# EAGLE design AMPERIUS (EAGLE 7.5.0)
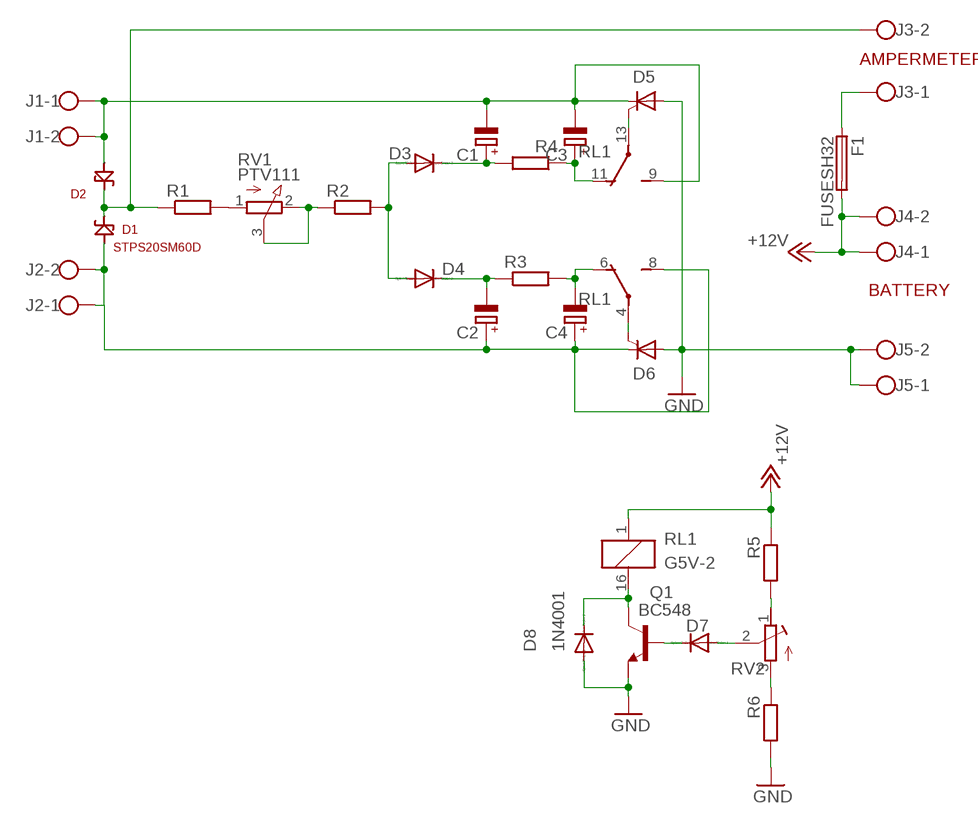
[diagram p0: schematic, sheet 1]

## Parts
C1  CPOL-EUE2.5-7  [E2,5-7]
C2  CPOL-EUE2.5-7  [E2,5-7]
C3  CPOL-EUE2.5-7  [E2,5-7]
C4  CPOL-EUE2.5-7  [E2,5-7]
D1  STPS20SM60D  [TO-220-2]
D2  STPS20SM60D  [TO-220-2]
D3  1N4148DO35-10  [DO35-10]
D4  1N4148DO35-10  [DO35-10]
D5  BTW58  [TO220CS]
D6  BTW58  [TO220CS]
D7  1N4148DO35-10  [DO35-10]
D8  1N4001  1N4004  [DO41-10]
F1  FUSESH32  [SH32]
J1  W237-102  [W237-102]
J2  W237-102  [W237-102]
J3  W237-102  [W237-102]
J4  W237-102  [W237-102]
J5  W237-102  [W237-102]
Q1  BC548  [TO92-EBC]
R1  R-EU_0207/10  [0207/10]
R2  R-EU_0207/10  [0207/10]
R3  R-EU_0207/10  [0207/10]
R4  R-EU_0207/10  [0207/10]
R5  R-EU_0207/10  [0207/10]
R6  R-EU_0207/10  [0207/10]
RL1  G5V-2  [G5V-2]
RV1  PTV111  [PTV111]
RV2  R-TRIMM-3386-F  [R-TRIMM-3386F]

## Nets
+12V: F1.2A J4.1 J4.2 R5.1 RL1.1
GND: D5.A D6.A D8.A J5.1 J5.2 Q1.E R6.2
N$1: D1.1(K) D2.1(K) J3.2 R1.1
N$2: C1.- C3.- D2.3(A) D5.C J1.1 J1.2 RL1.9(2:S)
N$3: C2.+ C4.+ D1.3(A) D6.C J2.1 J2.2 RL1.8(1:S)
N$4: R1.2 RV1.1(A)
N$5: R2.1 RV1.2(E) RV1.3(S)
N$6: D3.A D4.A R2.2
N$7: C1.+ D3.C R4.2
N$8: C2.- D4.C R3.1
N$9: F1.1A J3.1
N$10: D5.G RL1.13(2:P)
N$11: C4.- R3.2 RL1.6(1:O)
N$12: R5.2 RV2.1(A)
N$13: R6.1 RV2.3(E)
N$14: D7.A RV2.2(S)
N$15: D7.C Q1.B
N$16: C3.+ R4.1 RL1.11(2:O)
N$17: D8.C Q1.C RL1.16
N$19: D6.G RL1.4(1:P)

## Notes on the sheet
- AMPERMETER
- BATTERY

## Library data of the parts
C1-C4 = rcl:CPOL-EU: POLARIZED CAPACITOR, European symbol
D1 D2 = STPS20SM60D:STPS20SM60D: Diode Schottky 60V 20A Through Hole TO-220AC Check availability; AVAILABILITY: In Stock; CHECK_PRICES: https://www.snapeda.com/parts/STPS20SM60D/STMicroelectronics/view-part/?ref=eda; DESCRIPTION: Diode Schottky 60 V 20A Through Hole TO-220AC; MF: STMicroelectronics; MP: STPS20SM60D; PACKAGE: TO-220 STMicroelectronics; PRICE: None; PURCHASE-URL: https://www.snapeda.com/api/url_track_click_mouser/?unipart_id=727029&manufacturer=STMicroelectronics&part_name=STPS20SM60D&search_term=shottky diode 20a to-220; SNAPEDA_LINK: https://www.snapeda.com/parts/STPS20SM60D/STMicroelectronics/view-part/?ref=snap
D3 D4 D7 = diode:1N4148: DIODE
D5 D6 = triac:BTW58: THYRISTOR
D8 = diode:1N4004: DIODE
F1 = fuse:FUSE: Fuse; OC_FARNELL: unknown; OC_NEWARK: unknown
J1-J5 = con-wago-500:W237-102: WAGO SCREW CLAMP; MPN: 237-102; OC_FARNELL: unknown; OC_NEWARK: 70K9898
Q1 = transistor-npn:BC548*: NPN Transistor
R1-R6 = rcl:R-EU_: RESISTOR, European symbol
RL1 = relay:G5V-2: OMRON PCB Relay Source: http://www.omron.com/ecb/products/pdf/en-g5v2.pdf; MPN: G5V-2 5DC; OC_FARNELL: 9949488; OC_NEWARK: 78K5703
RV1 = pot:PTV111
RV2 = rcl:R-TRIMM-3386-F

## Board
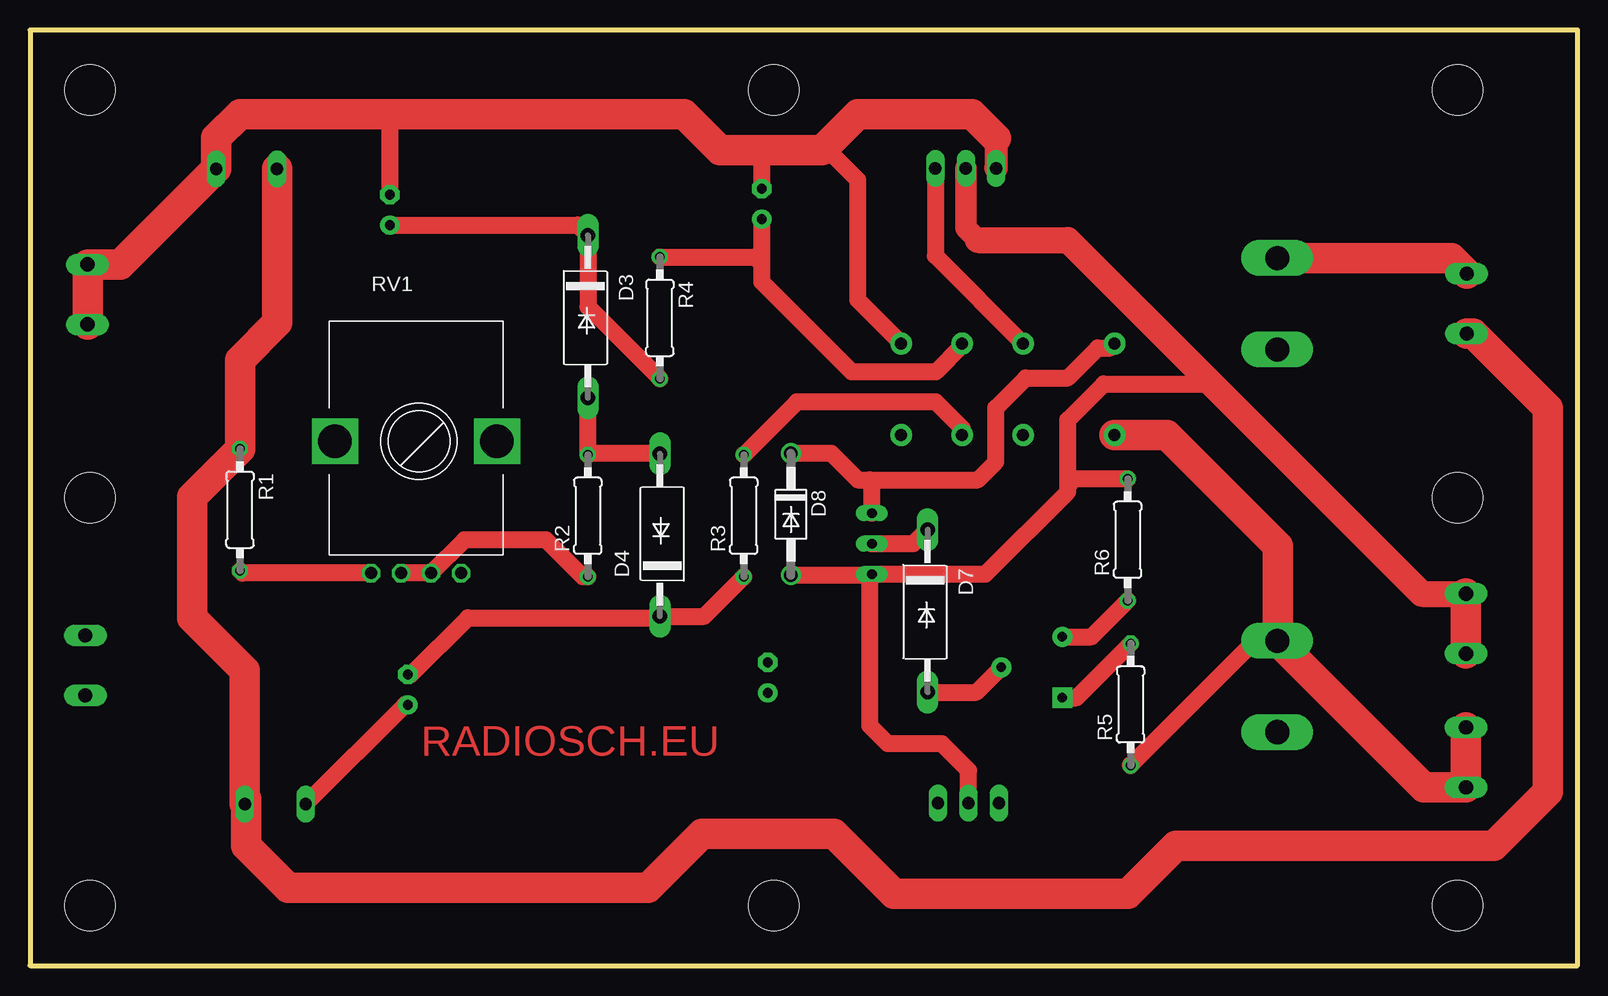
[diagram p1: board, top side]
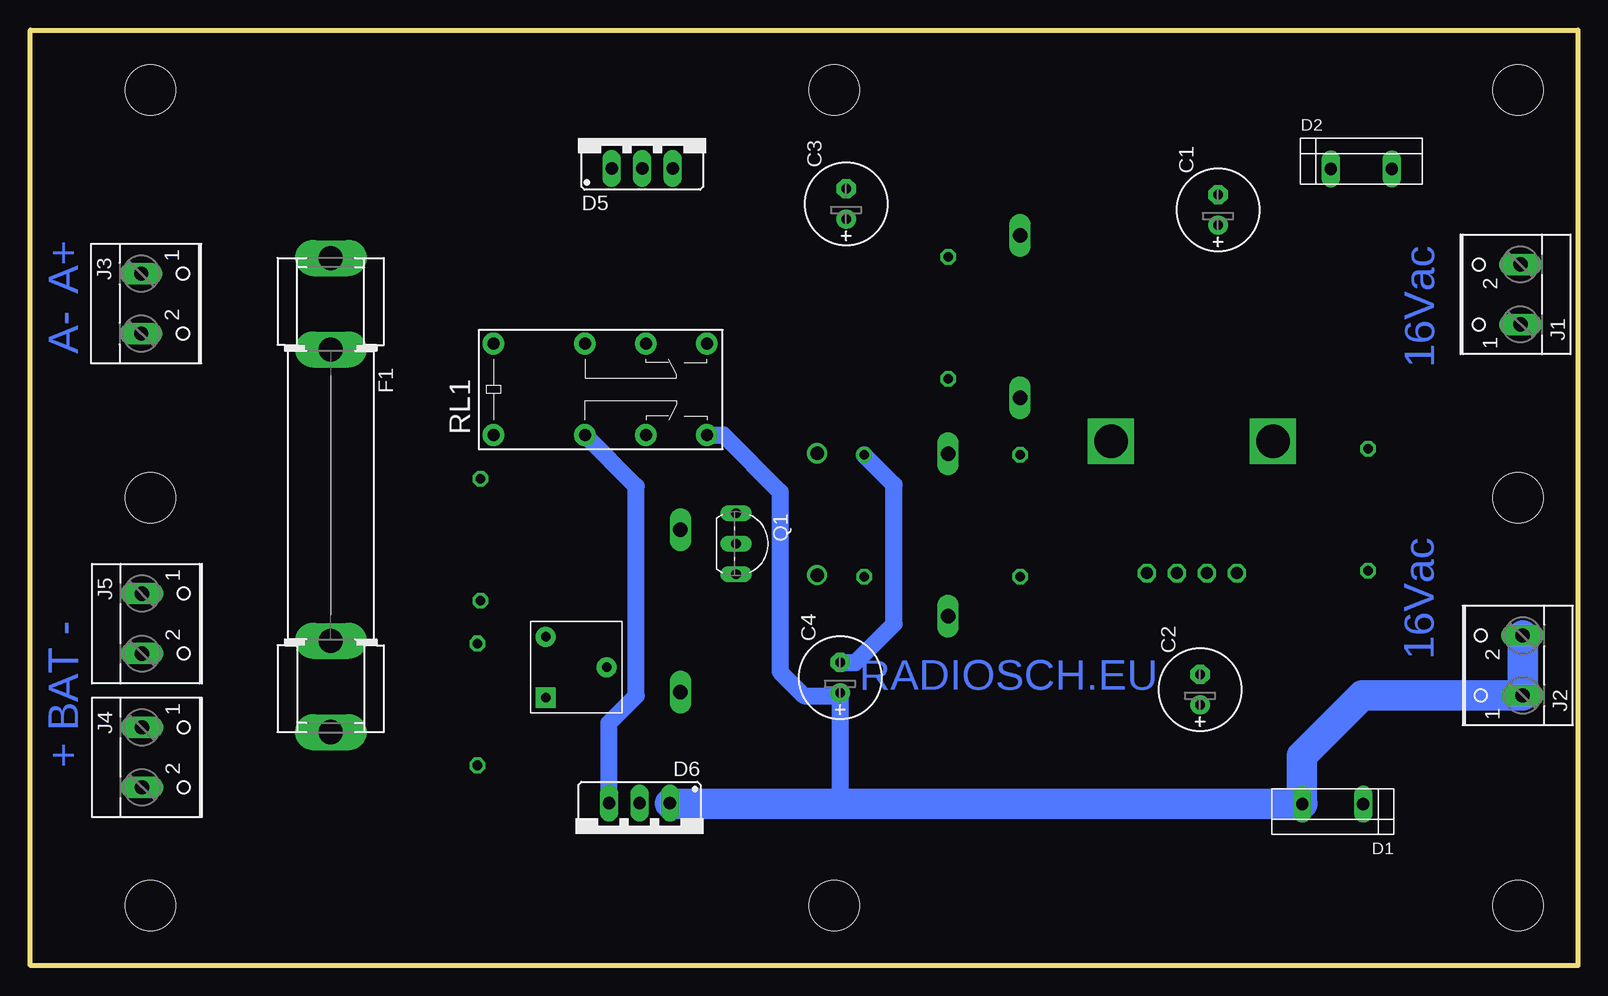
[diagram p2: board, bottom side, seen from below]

Size 129 x 78 mm. Coordinates in mm from the lower left corner, seen from the top.
Outline: 0,0 129,0 129,78 0,78 0,0
Copper layers (1*16): Top 0.035mm / dielectric 1.5mm / Bottom 0.035mm
Design rules "default": minimum track width 10mil, minimum drill 24mil, track to track 8mil, track to pad 8mil, pad to pad 8mil, via to via 8mil, smd to smd 8mil, copper to edge 40mil, drill to drill 8mil, minimum pad ring 10mil, minimum via ring 8mil, stop-mask expansion 4mil, vias tented up to drill 0mil, thermal gap 10mil
Holes 4.2 mm at 5,73 5,5 5,39 119,5 119,73 119,39 62,5 62,73

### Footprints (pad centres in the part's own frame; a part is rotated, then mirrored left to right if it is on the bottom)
E2,5-7 = drill 0.813 pad 1.6: + -1.27,0 | drill 0.813 pad 1.6 octagon: - 1.27,0
TO-220-2 = drill 1.016 long: 1 -2.54,0; 3 2.54,0
DO35-10 = drill 1.2 long: A 8.18,0; C -5.38,0
TO220CS = drill 1.016 long: A 0,-2.54; C -2.54,-2.54; G 2.54,-2.54
DO41-10 = drill 1.118: A 5.08,0; C -5.08,0
SH32 = drill 2.007 long: 1A -16.764,0; 1B -9.144,0; 2A 15.144,0; 2B 22.764,0
W237-102 = drill 1.194 long: 1 -2.5,-1.27; 2 2.5,-1.27
TO92-EBC = drill 0.813 long: B 0,-1.27; C -2.54,-1.27; E 2.54,-1.27
0207/10 = drill 0.813 octagon: 1 -5.08,0; 2 5.08,0
G5V-2 = drill 1 pad 1.8: 1 -8.89,-3.81; 4 -1.27,-3.81; 6 3.81,-3.81; 8 8.89,-3.81; 9 8.89,3.81; 11 3.81,3.81; 13 -1.27,3.81; 16 -8.89,3.81
PTV111 = drill 1 octagon: 1 3,-11; 2 8,-11; 3 5.5,-11; 4 10.5,-11 | drill 2.8 square: P$1 0,0; P$2 13.5,0
R-TRIMM-3386F = drill 0.8 pad 1.676 square: 1 0,0 | drill 0.8 pad 1.676: 2 5.08,2.54; 3 0,5.08

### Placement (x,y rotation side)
C1  30,63 90 bottom
C2  31.5,23 90 bottom
C3  61,63.5 90 bottom
C4  61.5,24 90 bottom
D1  20.45,13.46 180 bottom
D2  18.05,66.42 0 bottom
D3  46.5,55.5 270 top
D4  52.5,34.5 90 top
D5  78,69 0 bottom
D6  78.24,11 180 bottom
D7  74.82,30.97 270 top
D8  63.43,37.63 270 top
F1  103.97,42.22 270 bottom
J1  6.07,55.95 90 bottom
J2  5.88,25.02 90 bottom
J3  118.5,55.19 270 bottom
J4  118.43,17.35 270 bottom
J5  118.43,28.51 270 bottom
Q1  68.91,35.17 270 bottom
R1  17.5,38 270 top
R2  46.5,37.5 90 top
R3  59.5,37.5 90 top
R4  52.5,54 270 top
R5  91.75,21.76 90 top
R6  91.5,35.5 90 top
RL1  81.51,48.04 0 bottom
RV1  25.43,43.71 0 top
RV2  86.05,22.33 0 bottom

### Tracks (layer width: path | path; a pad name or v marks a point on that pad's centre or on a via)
+12V
  Top 1.422: R5.1 91.75,16.75 102,27 103.89,27 F1.2A
  Top 2.54: RL1.1 94.77,44.23 104,35 104,27.11 F1.2A 116.2,14.85 J4.2 J4.1
GND
  Top 1.422: Q1.E 79.63,32.63 86.5,39.5 86.5,40 | 86.5,40 86.5,45.5 89.5,48.5 98,48.5 98.25,48.75 | R6.2 87.08,40.58 86.5,40 | D6.A 78.24,16.26 76,18.5 71.5,18.5 70,20 70,32.45 Q1.E | D8.A 70.1,32.55 Q1.E
  Top 1.778: D5.A 78,61.5 79,60.5
  Top 2.184: 79,60.5 86.5,60.5 98.25,48.75 116,31 J5.1
  Top 2.54: J5.2 J5.1
N$1
  Top 2.54: D2.1 20.59,53.59 17.5,50.5 R1.1 13.5,39.08 13.5,29 17.91,24.59 17.91,14 | D1.1 17.91,14 | J3.2 120.31,52.69 126.5,46.5 126.5,14.5 122,10 95.5,10 91.5,6 72,6 67,11 56,11 51.5,6.5 21.5,6.5 18,10 18,13.91 17.91,14
N$2
  Top 1.422: 66.25,68.25 69,65.5 69,55.5 72.62,51.88 RL1.9 | C3.- 61,68 | C1.- 30,70.5 30.5,71
  Top 1.93: 80.5,69 80.5,66.5 D5.C
  Top 2.54: J1.1 J1.2 7.54,58.45 D2.3 15.51,69.01 17.5,71 30.5,71 54.5,71 57.5,68 61,68 66,68 66.25,68.25 69,71 78.5,71 80.5,69
N$3
  Top 1.422: C2.+ 31.26,21.73 D1.3
  Bottom 1.422: 61,13.46 61.5,13.96 C4.+ 61.73,22.5 64.5,22.5 66.5,24.5 66.5,39.5 71.23,44.23 RL1.8
  Bottom 2.54: J2.2 J2.1 17.98,22.52 23,17.5 D1.3 61,13.46 75.62,13.46 D6.C
N$4
  Top 1.422: RV1.1 17.71,32.71 R1.2
N$5
  Top 1.422: R2.1 46.08,32.42 43,35.5 36.22,35.5 RV1.2 RV1.3
N$6
  Top 1.422: D4.A 46.6,42.68 R2.2 D3.A
N$7
  Top 1.422: C1.+ 45.65,61.73 D3.C 46.5,54.92 R4.2
N$8
  Top 1.422: C2.- 31.77,24.27 36.5,29 52.38,29 D4.C 56.2,29.12 R3.1
N$9
  Top 2.54: F1.1A 118.48,58.98 J3.1
N$10
  Top 1.422: D5.G 75.46,59.17 RL1.13
N$11
  Top 1.422: RL1.6 77.7,44.8 75.5,47 63.92,47 R3.2
  Bottom 1.422: C4.- 60.23,25.27 57,28.5 57,40.08 R3.2
N$12
  Top 1.422: RV2.1 87.24,22.33 R5.2
N$13
  Top 1.422: RV2.3 88.49,27.41 R6.1
N$14
  Top 1.422: D7.A 78.89,22.79 RV2.2
N$15
  Top 1.422: Q1.B 73.64,35.17 D7.C
N$16
  Top 1.422: RL1.11 77.7,51.7 75.5,49.5 68.5,49.5 61,57 61,58.5 | 61,58.5 C3.+ | R4.1 60.42,59.08 61,58.5
N$17
  Top 1.422: D8.C 66.79,42.71 69,40.5 70,40.5 | 70,40.5 79,40.5 80.5,42 80.5,46.5 83,49 86.5,49 89,51.5 90.05,51.5 RL1.16 | Q1.C 70.18,40.32 70,40.5
N$19
  Bottom 1.422: D6.G 80.78,20.22 78.5,22.5 78.5,39.95 RL1.4

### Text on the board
Top: RADIOSCH.EU
Bottom: 16Vac | A+ | A- | 16Vac | RADIOSCH.EU | + BAT -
